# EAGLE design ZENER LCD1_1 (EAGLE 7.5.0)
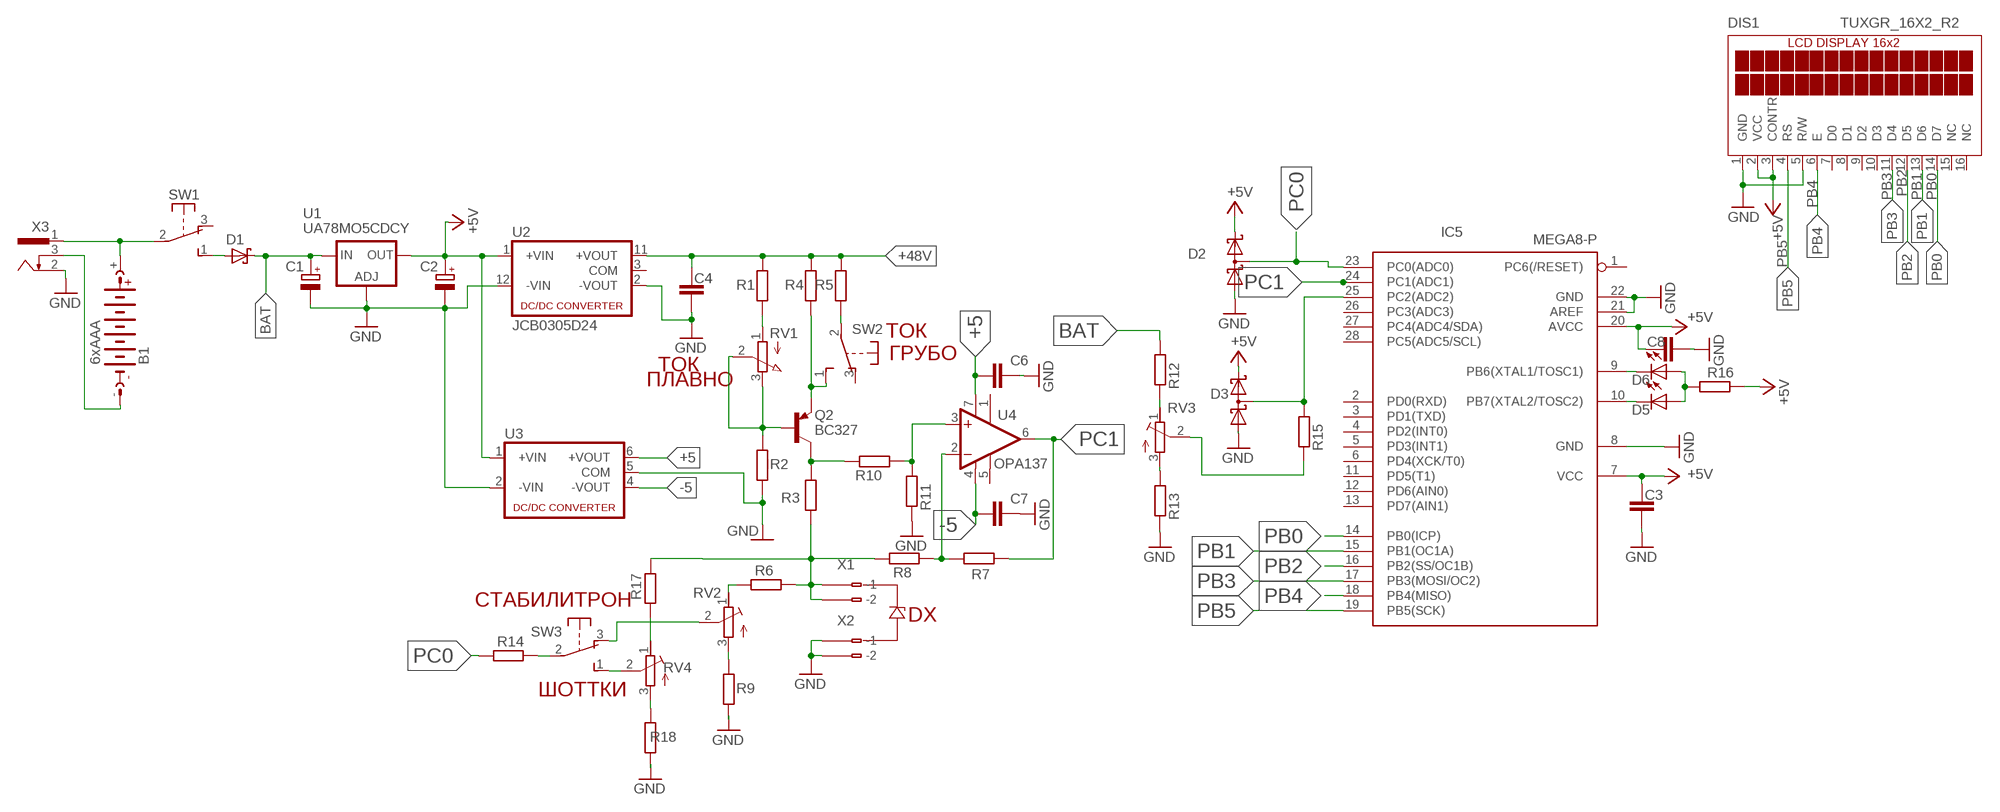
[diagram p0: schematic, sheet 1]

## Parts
B1  6xAAA  AB9V  [AB9V]
C1  CPOL-EUSMCC  [SMC_C]
C2  CPOL-EUSMCC  [SMC_C]
C3  C-EUC1206  [C1206]
C4  C-EUC1206  [C1206]
C6  C-EUC1206  [C1206]
C7  C-EUC1206  [C1206]
C8  C-EUC1206  [C1206]
D1  MBRS130LT3  [SMB]
D2  BAT54S  [SOT23]
D3  BAT54S  [SOT23]
D5  LED3MM  [LED3MM]
D6  LED3MM  [LED3MM]
DIS1  TUXGR_16X2_R2  [TUXGR_16X2_R2]
IC5  MEGA8-P  [DIL28-3]
Q2  BC327  [TO92]
R1  R-EU_R1206  [R1206]
R2  R-EU_R1206  [R1206]
R3  R-EU_R1206  [R1206]
R4  R-EU_R1206  [R1206]
R5  R-EU_R1206  [R1206]
R6  R-EU_R1206  [R1206]
R7  R-EU_R1206  [R1206]
R8  R-EU_R1206  [R1206]
R9  R-EU_R1206  [R1206]
R10  R-EU_R1206  [R1206]
R11  R-EU_R1206  [R1206]
R12  R-EU_R1206  [R1206]
R13  R-EU_R1206  [R1206]
R14  R-EU_R1206  [R1206]
R15  R-EU_R1206  [R1206]
R16  R-EU_R1206  [R1206]
R17  R-EU_R1206  [R1206]
R18  R-EU_R1206  [R1206]
RV1  PV09A  [PTV09]
RV2  R-TRIMM-3386-F  [R-TRIMM-3386F]
RV3  R-TRIMM-3386-F  [R-TRIMM-3386F]
RV4  R-TRIMM-3386-F  [R-TRIMM-3386F]
SW1  9077-1  [9077-1]
SW2  9077-1  [9077-1]
SW3  9077-1  [9077-1]
U1  UA78MO5CDCY  LD117AS33TR  [SOT223]
U2  JCB0305D24  [JCB0305D24]
U3  NMA  [NMA]
U4  OPA137  OPA131P  [DIL08]
X1  234-502  [234-502]
X2  234-502  [234-502]
X3  733980-62  [733980-62]

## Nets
+5: C6.2 U3.6(+VOUT) U4.7(V+)
+5V: C2.+ C3.2 C8.2 D2.2(C2) D3.2(C2) DIS1.2(VCC) DIS1.3(CONTR) IC5.7(VCC) IC5.20(AVCC) R16.2 U1.3(OUT) U2.1(+VIN) U3.1(+VIN)
+48V: C4.2 R1.2 R4.2 R5.2 U2.11(+VOUT)
-5: C7.2 U3.4(-VOUT) U4.4(V-)
BAT: C1.+ D1.C R12.1 U1.1(IN)
GND: C1.- C2.- C3.1 C4.1 C6.1 C7.1 C8.1 D2.1(A1) D3.1(A1) DIS1.1(GND) DIS1.5(R/W) IC5.8(GND) IC5.21(AREF) IC5.22(GND) R2.1 R9.1 R11.2 R13.2 R18.1 U1.2(ADJ) U2.2(-VOUT) U2.12(-VIN) U3.2(-VIN) U3.5(COM) X2.B1(B-1) X2.B2(B-2) X3.2
N$1: Q2.3(C) R3.2 R10.2
N$2: Q2.2(B) R2.2 RV1.2(S) RV1.3(E)
N$3: R1.1 RV1.1(A)
N$4: Q2.1(E) R4.1 SW2.1(S)
N$5: D6.K(C) IC5.9(PB6(XTAL1/TOSC1))
N$6: R5.1 SW2.2(P)
N$7: R9.2 RV2.3(E)
N$8: R6.2 RV2.1(A)
N$9: R18.2 RV4.3(E)
N$10: R7.2 R8.1 U4.2(-IN)
N$11: R10.1 R11.1 U4.3(+IN)
N$12: D1.A SW1.1(S)
N$13: D3.3(C1A2) IC5.25(PC2(ADC2)) R15.1
N$14: R15.2 RV3.2(S)
N$15: R13.1 RV3.3(E)
N$16: R12.2 RV3.1(A)
N$17: R3.1 R6.1 R8.2 R17.1 X1.B1(B-1) X1.B2(B-2)
N$18: D5.K(C) IC5.10(PB7(XTAL2/TOSC2))
N$19: D5.A D6.A R16.1
N$20: B1.- X3.3
N$21: R17.2 RV4.1(A)
N$23: RV4.2(S) SW3.1(S)
N$25: R14.1 SW3.2(P)
N$26: RV2.2(S) SW3.3(O)
N$41: B1.+ SW1.2(P) X3.1
PB0: DIS1.14(D7) IC5.14(PB0(ICP))
PB1: DIS1.13(D6) IC5.15(PB1(OC1A))
PB2: DIS1.12(D5) IC5.16(PB2(SS/OC1B))
PB3: DIS1.11(D4) IC5.17(PB3(MOSI/OC2))
PB4: DIS1.6(E) IC5.18(PB4(MISO))
PB5: DIS1.4(RS) IC5.19(PB5(SCK))
PC0: D2.3(C1A2) IC5.23(PC0(ADC0)) R14.2
PC1: IC5.24(PC1(ADC1)) R7.1 U4.6(OUT)
Unconnected: DIS1.7(D0) DIS1.8(D1) DIS1.9(D2) DIS1.10(D3) DIS1.15(NC) DIS1.16(NC) IC5.1(PC6(/RESET)) IC5.2(PD0(RXD)) IC5.3(PD1(TXD)) IC5.4(PD2(INT0)) IC5.5(PD3(INT1)) IC5.6(PD4(XCK/T0)) IC5.11(PD5(T1)) IC5.12(PD6(AIN0)) IC5.13(PD7(AIN1)) IC5.26(PC3(ADC3)) IC5.27(PC4(ADC4/SDA)) IC5.28(PC5(ADC5/SCL)) SW1.3(O) SW2.3(O) U2.3(COM) U4.1(TRIM1) U4.5(TRIM2) X1.A1(-1) X1.A2(-2) X2.A1(-1) X2.A2(-2)

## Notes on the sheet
- ТОК
- ГРУБО
- ТОК
- ПЛАВНО
- СТАБИЛИТРОН
- DX
- ШОТТКИ

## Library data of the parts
B1 = battery:AB9V: 9-V BATTERY CLIP
C1 C2 = rcl:CPOL-EU: POLARIZED CAPACITOR, European symbol
C3 C4 C6-C8 = rcl:C-EU: CAPACITOR, European symbol
D1 = diode:MBRS130LT3: Schottky Power Rectifier
D2 D3 = diode:BAT54S: Schottky Diodes Pin connection corrected 2011-05-04 Source: Fairchild .. BAT54.pdf
D5 D6 = led:LED: LED
DIS1 = display-lcd:TUXGR_16X2_R2: Tuxgraphics LCD display 16x2 characters reflective, without background light Source: tuxgr_12x2_r2.pdf; OC_FARNELL: unknown; OC_NEWARK: unknown
IC5 = atmel:MEGA8-P: MICROCONTROLLER 8 Kbytes FLASH, 1 kbytes SRAM, 512 bytes EEPROM, USART, 4-channel 10 bit ADC, 2-channel 8 bit ADC Pin compatible with Atmega48, ATMega88, ATMega168 Source: avr.lbr; OC_FARNELL: unknown; OC_NEWARK: unknown
Q2 = transistor-pnp:BC327: PNP Transistor
R1-R18 = rcl:R-EU_: RESISTOR, European symbol
RV1 = pot:PV09A
RV2-RV4 = rcl:R-TRIMM-3386-F
SW1-SW3 = switch-misc:9077-1: MARQUARDT SWITCH 9077.0100 Distributor: Buerklin
U1 = v-reg:LD117A?*: Low drop fixed and adjustable positive voltage regulators 1 A Source: http://www.st.com/stonline/products/literature/ds/7194/ld1117axx.pdf
U2 = dc-dc-converter:JCB0305D24: Isolated Board Mount DC/DC Converter, 2:1 Input, ITE, 2 Output, 3 W, 24 V, 63 mA, -24 V
U3 = dc-dc-converter:NMA: DC-DC CONVERTER; MF: C & D TECHNOLOGIES, INC; MPN: NMA0515SC; OC_FARNELL: 1021434; OC_NEWARK: 61K3064
U4 = burr-brown:OPA131: Operational Amplifiers General Purpose FET-Input; OC_FARNELL: unknown; OC_NEWARK: unknown
X1 X2 = con-wago:234-502: WAGO Cage Clamp; MPN: 234-502; OC_FARNELL: 1777106; OC_NEWARK: 28K9105
X3 = con-conrad:73398?: FEMALE PRINT CONNECTOR Niedervolt-Steckverbinder Distributor Conrad

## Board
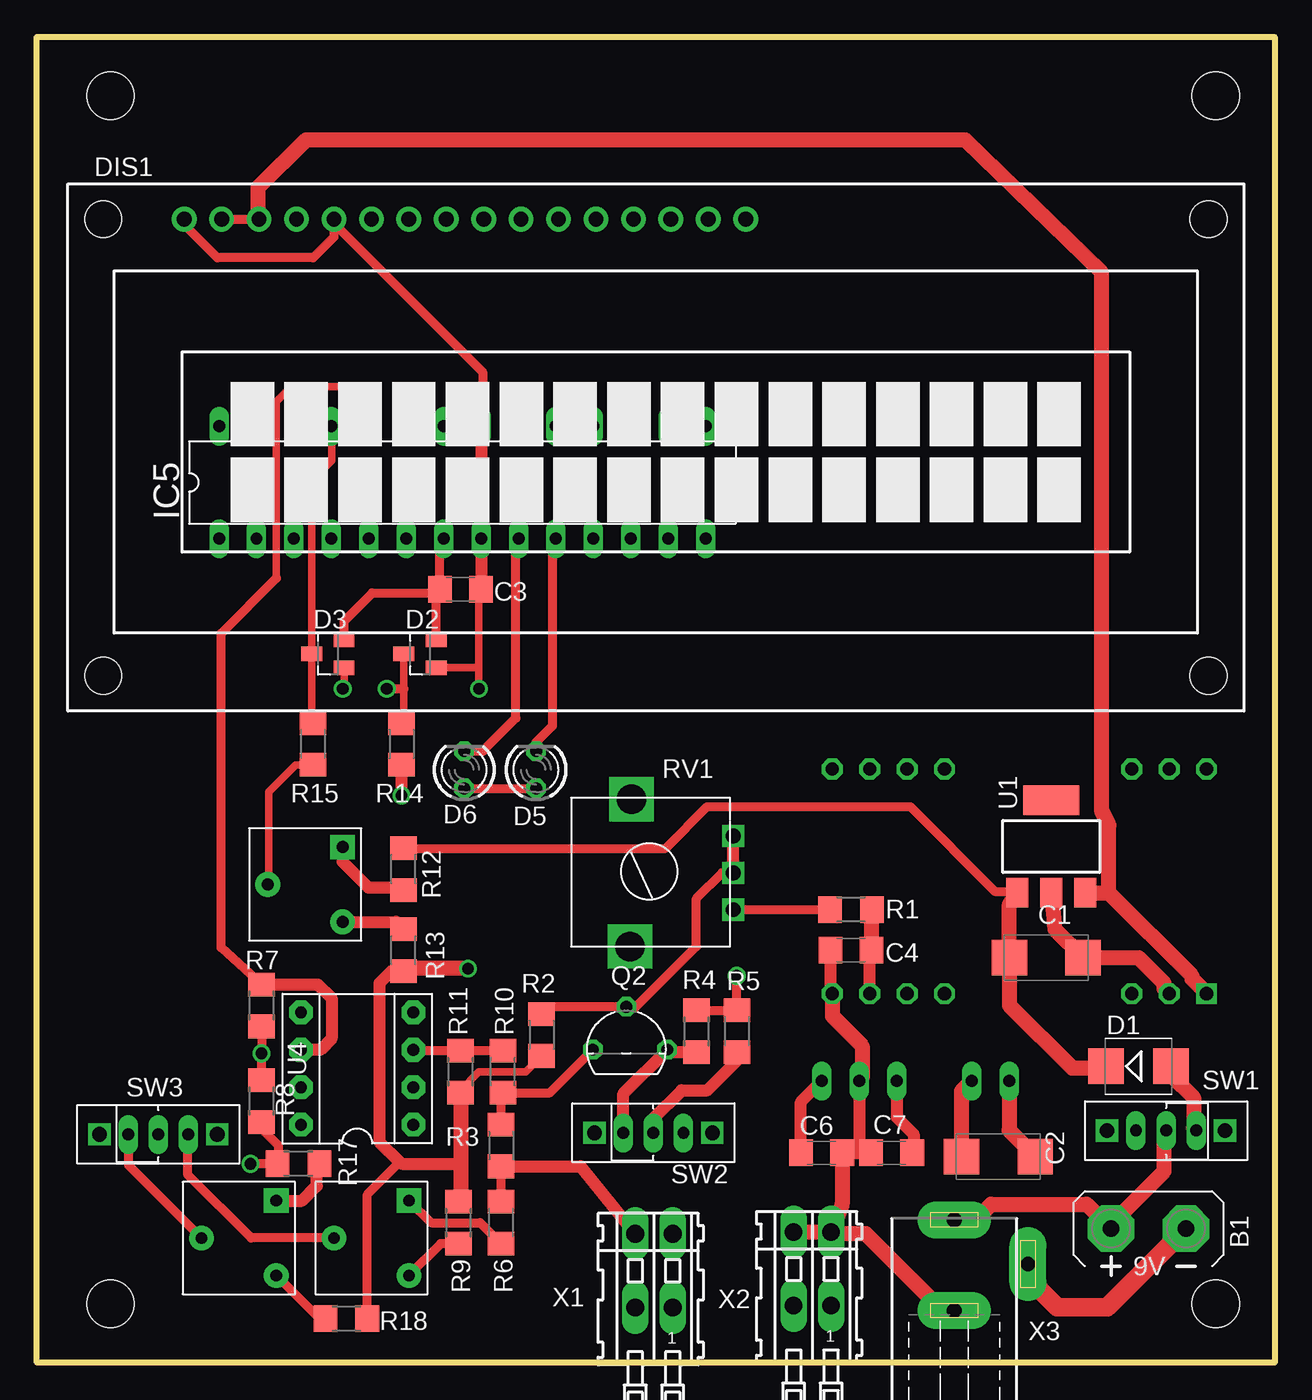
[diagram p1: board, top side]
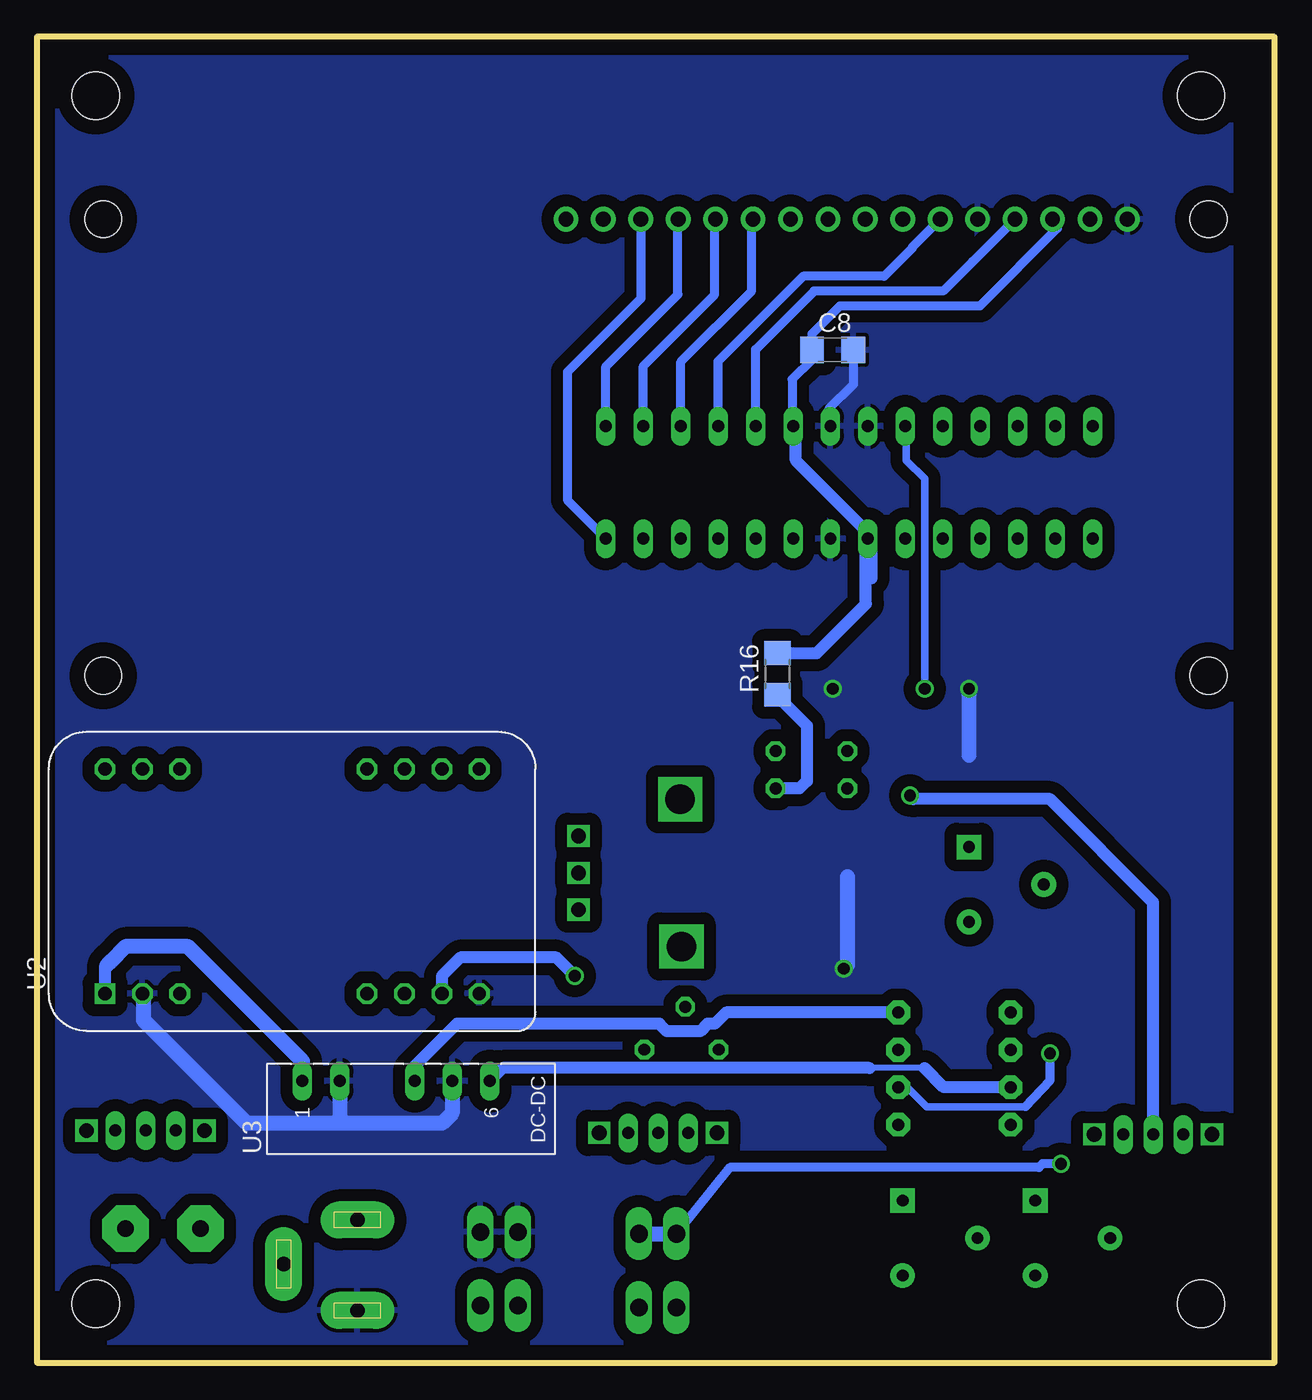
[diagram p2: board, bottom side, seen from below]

Size 84 x 90 mm. Coordinates in mm from the lower left corner, seen from the top.
Outline: 0,0 0,90 84,90 84,0 0,0
Copper layers (1*16): Top 0.035mm / dielectric 1.5mm / Bottom 0.035mm
Design rules "default *": minimum track width 10mil, minimum drill 24mil, track to track 6mil, track to pad 6mil, pad to pad 6mil, via to via 8mil, smd to smd 8mil, copper to edge 40mil, drill to drill 8mil, minimum pad ring 10mil, minimum via ring 8mil, stop-mask expansion 4mil, vias tented up to drill 0mil, thermal gap 10mil
Holes 3.2 mm at 5,4 80,4 5,86 80,86

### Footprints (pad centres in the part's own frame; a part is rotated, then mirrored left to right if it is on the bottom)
AB9V = drill 1.118 pad 3.15 octagon: + 0,2.54; - 0,-2.54
SMC_C = smd 2.4 x 2.4: + -2.5,0; - 2.5,0
C1206 = smd 1.6 x 1.8: 1 -1.4,0; 2 1.4,0
SMB = smd 2.4 x 2.4: A 2.2,0; C -2.2,0
SOT23 = smd 1 x 1.4: 1 -0.95,-1.1; 2 0.95,-1.1; 3 0,1.1
LED3MM = drill 0.813 octagon: A -1.27,0; K 1.27,0
TUXGR_16X2_R2 = drill 1 pad 1.676: 1 -32,15.5; 2 -29.46,15.5; 3 -26.92,15.5; 4 -24.38,15.5; 5 -21.84,15.5; 6 -19.3,15.5; 7 -16.76,15.5; 8 -14.22,15.5; 9 -11.68,15.5; 10 -9.14,15.5; 11 -6.6,15.5; 12 -4.06,15.5; 13 -1.52,15.5; 14 1.02,15.5; 15 3.56,15.5; 16 6.1,15.5 | hole 2.5: -37.5,-15.5; 37.5,-15.5; -37.5,15.5; 37.5,15.5
DIL28-3 = drill 0.813 long: 1 -16.51,-3.81; 2 -13.97,-3.81; 3 -11.43,-3.81; 4 -8.89,-3.81; 5 -6.35,-3.81; 6 -3.81,-3.81; 7 -1.27,-3.81; 8 1.27,-3.81; 9 3.81,-3.81; 10 6.35,-3.81; 11 8.89,-3.81; 12 11.43,-3.81; 13 13.97,-3.81; 14 16.51,-3.81; 15 16.51,3.81; 16 13.97,3.81; 17 11.43,3.81; 18 8.89,3.81; 19 6.35,3.81; 20 3.81,3.81; 21 1.27,3.81; 22 -1.27,3.81; 23 -3.81,3.81; 24 -6.35,3.81; 25 -8.89,3.81; 26 -11.43,3.81; 27 -13.97,3.81; 28 -16.51,3.81
TO92 = drill 0.813 octagon: 1 2.77,0; 2 0,2.905; 3 -2.27,0
R1206 = smd 1.6 x 1.803: 1 -1.422,0; 2 1.422,0
PTV09 = drill 1 square: 1 -2.5,0; 2 0,0; 3 2.5,0 | drill 2 square: P$4 -5,7; P$5 5,6.9
R-TRIMM-3386F = drill 0.8 pad 1.676 square: 1 0,0 | drill 0.8 pad 1.676: 2 5.08,2.54; 3 0,5.08
9077-1 = drill 0.813 long: 1 -2.04,-1.016; 2 0,-1.016; 3 2.04,-1.016 | drill 1 square: P$1 -4,-1; P$2 4,-1
SOT223 = smd 1.5 x 2: 1 -2.3,-3.15; 2 0,-3.15; 3 2.3,-3.15 | smd 3.8 x 2: 4 0,3.15
JCB0305D24 = drill 0.9 square: 1 0,0 | drill 0.9 octagon: 2 2.54,0; 3 5.08,0; 9 17.78,0; 10 20.32,0; 11 22.86,0; 12 25.4,0; 13 25.4,15.24; 14 22.86,15.24; 15 20.32,15.24; 16 17.78,15.24; 22 5.08,15.24; 23 2.54,15.24; P$8 0,15.24
NMA = drill 0.813 long: 1 0,6.35; 2 0,3.81; 4 0,-1.27; 5 0,-3.81; 6 0,-6.35
DIL08 = drill 0.813 pad 1.6 octagon: 1 -3.81,-3.81; 2 -1.27,-3.81; 3 1.27,-3.81; 4 3.81,-3.81; 5 3.81,3.81; 6 1.27,3.81; 7 -1.27,3.81; 8 -3.81,3.81
234-502 = drill 1.2 long: A1 -1.27,2.5; A2 1.27,2.5; B1 -1.27,-2.5; B2 1.27,-2.5
733980-62 = drill 1 pad 2.5 long: 1 0,8.57; 2 0,2.42; 3 5,5.57

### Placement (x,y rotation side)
B1  75.44,9.1 90 top
C1  68.5,27.5 0 top
C2  65.25,14 180 top
C3  28.75,52.5 180 top
C4  55.25,28 0 top
C6  53.25,14.25 180 top
C7  58,14.25 0 top
C8  30,68.75 180 bottom
D1  74.75,20.12 0 top
D2  26,48.12 90 top
D3  19.75,48.12 90 top
D5  33.88,40.25 90 top
D6  29,40.25 90 top
DIS1  42,62.12 0 top
IC5  28.88,59.75 0 top
Q2  40,21.25 0 top
R1  55.25,30.75 0 top
R2  34.25,22.25 90 top
R3  31.5,14.75 90 top
R4  44.75,22.5 90 top
R5  47.5,22.5 90 top
R6  31.5,9.5 270 top
R7  15.25,24.25 270 top
R8  15.25,17.75 270 top
R9  28.62,9.5 270 top
R10  31.62,19.75 270 top
R11  28.75,19.75 270 top
R12  24.88,33.5 270 top
R13  24.88,28 270 top
R14  24.75,42 90 top
R15  18.75,42 270 top
R16  33.75,46.75 90 bottom
R17  17.75,13.5 0 top
R18  21,3 180 top
RV1  47.25,33.25 90 top
RV2  25.25,11 180 top
RV3  20.75,35 180 top
RV4  16.25,11 180 top
SW1  76.62,14.75 180 top
SW2  41.84,16.61 0 top
SW3  8.25,16.5 0 top
U1  68.83,35.05 0 top
U2  79.38,25.05 0 bottom
U3  59.62,19.12 90 bottom
U4  21.73,19.96 90 top
X1  41.88,6.25 180 top
X2  52.62,6.38 180 top
X3  62.25,1.12 0 top

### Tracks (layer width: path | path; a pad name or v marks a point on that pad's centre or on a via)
+5
  Top 0.813: C6.2 51.85,17.7 U3.6
  Bottom 0.4: 23.75,20 27.5,20
  Bottom 0.813: U4.7 22.45,18.7 23.75,20 | 27.5,20 52.4,20 U3.6
+5V
  Top 0.61: D3.2 20.85,50.35 22.75,52.25 27.1,52.25 | D2.2 27.1,52.25 | 27.1,52.25 C3.2 27.35,55.69 IC5.7 | DIS1.2 DIS1.3
  Top 1.016: U3.1 65.97,15.78 C2.+ | U1.3 72.75,31.89 | DIS1.3 15,77.7 15,79.75 18.25,83 63,83 72.25,74 72.25,37.5 72.75,36.5 72.75,31.89 | U2.1 78.39,26.04 78.39,26.25 72.75,31.89
  Bottom 0.61: IC5.20 32.75,63.62 32.75,66.75 31.4,68.1 C8.2 31.4,69.85 29.5,71.75 20,71.75 14.75,77 14.75,77.3 DIS1.3
  Bottom 0.813: IC5.20 32.5,63.38 32.5,61.25 27.61,56.35 IC5.7 27.35,55.69 27.35,55.5 | 27.35,53.25 27.35,55.5 | R16.2 31.08,48.17 27.75,51.5 27.75,55.1 27.35,55.5 | U2.1 79.38,26.88 79,27.25
  Bottom 1.016: U3.1 65.97,20.48 73.75,28.25 78,28.25 79,27.25 79.25,27
+48V  (via drill 0.8)
  Top 0.61: R4.2 R5.2 v47.5,26.25
  Top 0.813: U2.11 56.52,27.86 C4.2
  Top 1.016: C4.2 56.65,30.73 R1.2
  Bottom 0.813: v47.5,26.25 48.75,27.5 55.27,27.5 56.52,26.25 U2.11
-5
  Top 0.813: U3.4 58.35,16.64 59.5,15.5 59.5,14.35 C7.2
  Bottom 0.813: U4.4 37.23,23.77 38,23 38.5,23 39,22.5 41.25,22.5 41.75,23 55.5,23 58.5,20 58.5,19.27 U3.4
BAT
  Top 0.61: R12.1 42.67,34.92 45.5,37.75 59.25,37.75 65,32 66.68,32 U1.1
  Top 1.016: D1.C 72.42,20 70.25,20 66,24.25 C1.+ 66,31.11 U1.1
GND  (via drill 0.8)
  Top 0.5: R11.2 28.75,18.5 30,19.75 33.17,19.75 R2.1 | D3.1 20.85,45.85 v20.75,45.75 | v30,45.75 30,47 | 30,47 30,52.35 C3.1 | D2.1 29.82,47.17 30,47
  Top 0.61: IC5.21 30.25,63.66 30.25,67.25 20.16,77.34 DIS1.5 20.16,76.41 18.75,75 12.25,75 10.25,77 10.25,77.38 DIS1.1 | R18.1 22.42,11.42 24.62,13.62
  Top 0.813: C4.1 53.85,25.18 U2.12 | C6.1 55.75,14.25 | 55.75,14.25 C7.1 | U3.5 55.81,14.31 55.75,14.25 | R13.2 24.08,26.58 23.25,25.75 23.25,15 24.62,13.62 24.75,13.5 28.5,13.5 28.75,13.25 | C3.1 IC5.8 IC5.21
  Top 1.016: U2.12 53.98,23.52 56,21.5 56,19.31 U3.5 | C2.- 62.75,18.44 U3.2 | U1.2 69.08,29.41 C1.- 74.75,27.5 76.5,25.75 76.5,25.39 U2.2 | R11.2 28.75,13.25 28.75,11.5 28.25,11 28.55,11 R9.1 | X3.2 61.45,3.54 56.25,8.75 54.65,8.75 X2.B1 | X2.B2 X2.B1 | C6.1 54.65,10.76 X2.B1 | v29.25,26.75 25.05,26.75 R13.2
  Bottom 0.61: C8.1 28.6,66.4 30.25,64.75 30.25,63.66 IC5.21
  Bottom 1.016: U3.5 55.81,16.93 56.5,16.25 63.25,16.25 | 63.25,16.25 69.75,16.25 76.75,23.25 76.75,24.97 U2.2 | U3.2 63.44,16.43 63.25,16.25 | v20.75,45.75 20.75,41.25 | 29,33 29,27 v29.25,26.75
  pour Bottom (isolate 0.813): 3,89 83.5,89 83.5,0.75 3,0.75
N$1
  Top 0.61: Q2.3 34.81,18.33 R10.2 31.5,18.2 R3.2
N$2
  Top 0.61: R2.2 34.73,24.16 Q2.2 40.66,24.16 44.75,28.25 44.75,31.5 46.5,33.25 RV1.2
  Top 0.813: RV1.2 RV1.3
N$3
  Top 0.61: R1.1 RV1.1
N$4
  Top 0.813: R4.1 42.94,21.08 Q2.1 39.8,18.28 SW2.1
N$5
  Top 0.61: D6.K 30.27,41.52 32.5,43.75 32.5,55.76 IC5.9
N$6
  Top 0.813: SW2.2 41.84,16.59 43.75,18.5 45.5,18.5 47.5,20.5 R5.1
N$7
  Top 0.61: R9.2 27.41,8.08 RV2.3
N$8
  Top 0.61: RV2.1 26.75,9.5 30.08,9.5 R6.2
N$9
  Top 0.61: R18.2 19.17,3 RV4.3
N$10  (via drill 0.8)
  Top 0.61: R7.2 v15.25,21 R8.1
  Bottom 0.5: U4.2 24.95,18.7 23.62,17.38 16.92,17.38
  Bottom 0.61: 16.92,17.38 R8.1 v15.25,21
N$11
  Top 0.61: R10.1 R11.1 25.61,21.17 U4.3
N$12
  Top 1.016: D1.A 76.95,19.55 78.5,18 78.5,15.93 SW1.1
N$13
  Top 0.5: IC5.25 20,63.55 20,61.25 18.65,59.9 D3.3 18.65,43.52 R15.1
N$14
  Top 0.5: R15.2 17.58,40.58 15.75,38.75 15.75,32.54 RV3.2
N$15
  Top 0.813: RV3.3 24.38,29.92 R13.1
N$16
  Top 0.813: RV3.1 20.75,34 22.5,32.25 24.7,32.25 R12.2
N$17  (via drill 0.8)
  Top 0.61: R6.1 R3.1 | v14.5,13.5 R17.1 16.38,13.55 16.38,14.75 15.25,15.88 R8.2
  Top 0.813: R3.1 36.9,13.33 X1.B2
  Bottom 0.61: X1.B2 36.98,13.25 16,13.25 15.75,13.5 v14.5,13.5
  Bottom 1.016: X1.B1 X1.B2
N$18
  Top 0.61: D5.K 33.88,42.12 35,43.25 35,55.72 IC5.10
N$19
  Top 0.61: D6.A D5.A
  Bottom 0.813: R16.1 33.75,45.25 31.75,43.25 31.75,39.48 32.25,38.98 D5.A
N$20
  Top 1.27: X3.3 67.25,5.75 69.25,3.75 72.63,3.75 B1.-
N$21
  Top 0.813: RV4.1 18,11 19,12 19,13.33 R17.2
N$23
  Top 0.61: SW3.1 6.21,13.42 RV4.2
N$25  (via drill 0.8)
  Top 0.813: v24.75,38.5 R14.1
  Bottom 0.813: SW3.2 8.25,31.25 15.25,38.25 24.5,38.25 v24.75,38.5
N$26
  Top 0.61: RV2.2 14.54,8.46 10.25,12.75 10.25,15.44 SW3.3
N$41
  Top 1.016: SW1.2 76.5,15.64 76.5,13 72.89,9.39 B1.+ 71.24,10.75 64.75,10.75 63.7,9.7 X3.1
PB0
  Bottom 0.61: DIS1.14 43.02,72.23 48,67.25 48,58.55 IC5.14
PB1
  Bottom 0.61: IC5.15 45.38,67.61 40.5,72.5 40.5,77.61 DIS1.13
PB2
  Bottom 0.61: IC5.16 42.84,67.66 38,72.5 38,77.56 DIS1.12
PB3
  Bottom 0.61: IC5.17 40.3,67.94 35.5,72.75 35.5,77.53 DIS1.11
PB4
  Bottom 0.61: IC5.18 37.77,67.98 32,73.75 26.5,73.75 24.57,75.67 24.57,75.75 DIS1.6
PB5
  Bottom 0.61: IC5.19 35.23,68.78 31.25,72.75 22.5,72.75 20.5,74.75 DIS1.4
PC0  (via drill 0.8)
  Top 0.5: D2.3 24.9,45.75 24.9,43.57 R14.2
  Top 0.61: D2.3 24.88,48.12 | v23.75,45.75 24.9,45.75
  Bottom 0.5: v23.75,45.75 23.75,60 25,61.25 25,63.49 IC5.23
PC1
  Top 0.5: 16.25,53.25 16.25,65.25 17.25,66.25 21.25,66.25 22.5,65 22.5,63.59 IC5.24
  Top 0.61: 16.25,53.25 12.5,49.5 12.5,28.17 R7.1
  Top 0.813: R7.1 19.08,25.67 20,24.75 20,22 19.25,21.25 17.94,21.25 U4.6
